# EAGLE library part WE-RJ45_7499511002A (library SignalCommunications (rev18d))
WE-RJ45 LAN Transformer Order Code 7499511002A Design THT xBase-T 10/100/1000 Base-T Ports 1x1 Application Standard Tab Position UP/DOWN LED (Left-Right) No EMI Fingers No Details see: http://katalog.we-online.de/en/pbs/WE-LAN-RJ45 Created by Yingchun Shan 2016 (C) Wurth Elektronik
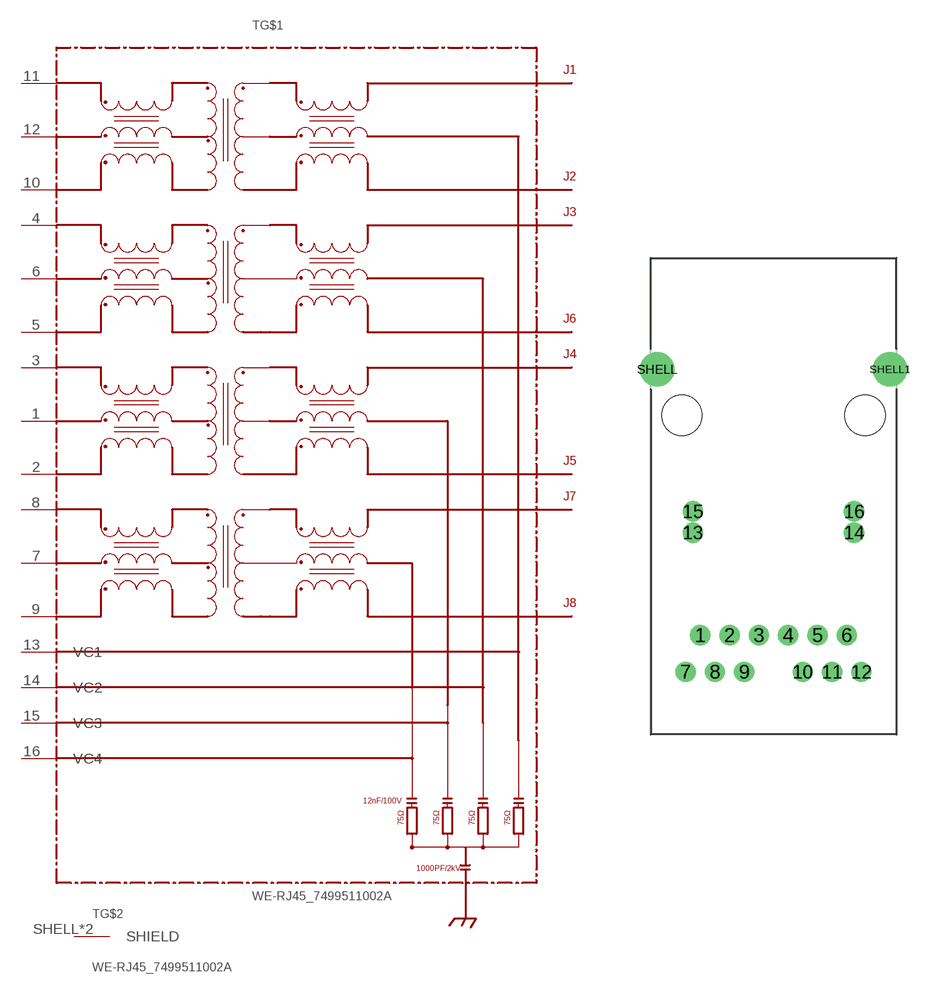
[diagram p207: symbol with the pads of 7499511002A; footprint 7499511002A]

Designator prefix T; gates G$1=7499511002A G$2=SHIELD

## WE-RJ45_7499511002A  [7499511002A]
1  G$1:P1
2  G$1:P2
3  G$1:P3
4  G$1:P4
5  G$1:P5
6  G$1:P6
7  G$1:P7
8  G$1:P8
9  G$1:P9
10  G$1:P10
11  G$1:P11
12  G$1:P12
13  G$1:VC1
14  G$1:VC2
15  G$1:VC3
16  G$1:VC4
SHELL  G$2:SHIELD  pas
SHELL1  G$2:SHIELD  pas

## Footprint 7499511002A (pad centres in mm)
drill 0.9: 1 -5.075,-15.24; 2 -3.045,-15.24; 3 -1.015,-15.24; 4 1.015,-15.24; 5 3.045,-15.24; 6 5.075,-15.24; 7 -6.09,-17.78; 8 -4.06,-17.78; 9 -2.03,-17.78; 10 2.03,-17.78; 11 4.06,-17.78; 12 6.09,-17.78; 13 -5.59,-8.13; 14 5.59,-8.13; 15 -5.59,-6.66; 16 5.59,-6.66
drill 1.6: SHELL -8.065,3.18; SHELL1 8.065,3.18
hole 2.8 at -6.35,0
hole 2.8 at 6.35,0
